(* Logix 5000 AddOnInstructionDefinition export HI6501_HMI_AOI_V1_2; software revision 30.00 *)

ADD_ON_INSTRUCTION HI6501_HMI_AOI_V1_2   (* revision 1.0 *)
VAR_IN_OUT
   From_Indicator : _0102:Hardy6500Series_3459222C:I:0; {required}   // Inputs from Hardy indicator
   To_Indicator : _0102:Hardy6500Series_B3FC222E:O:0; {required}   // Outputs to Hardy indicator
END_VAR
VAR_INPUT
   Remote_Zero : BOOL;   // Remote zero input signal
   Remote_Tare : BOOL;   // Remote tare input signal
   Mode_Select_PB : BOOL;   // Gross Net mode toggle select from faceplate
END_VAR
VAR_OUTPUT
   Gross_Mode_To_FP : BOOL; {access Read Only}   // Gross weight display mode output to faceplate
   Net_Mode_To_FP : BOOL; {access Read Only}   // Net weight display mode output to faceplate
   Gross_Weight : REAL; {access Read Only, visible}   // Gross weight
   Net_Weight : REAL; {access Read Only, visible}   // Net weight
   Alarm : BOOL; {access Read Only, visible}   // Alarm output
   Decimal_Point_To_FP : SINT;   // Decimal point parameter input value to faceplate
   Grads_To_FP : SINT;   // Graduations parameter input value to faceplate
   Unit_To_FP : SINT;   // Units parameter input value to faceplate
   Waversaver_To_FP : SINT;   // WAVERSAVER parameter input value to faceplate
   Num_Averages_To_FP : INT;   // Number of averages parameter input value to faceplate
   Loadcell_Sensitivity_To_FP : INT;   // Load cell sensitivity parameter input value to faceplate
   AutoZero_To_FP : INT;   // Auto zero parameter input value to faceplate
   AutoZero_Tol_To_FP : REAL;   // Auto zero tolerance parameter input value to faceplate
   Gravity_Correction_To_FP : REAL;   // Gravity correction parameter input value to faceplate
   Motion_Tol_To_FP : REAL;   // Motion tolerance parameter input value to faceplate
   Zero_Tol_To_FP : REAL;   // Zero tolerance parameter input value to faceplate
   Tare_Weight_To_FP : REAL;   // Tare weight parameter input value to faceplate
   Reference_Weight_To_FP : REAL;   // Reference weight parameter input value to faceplate
   Span_Weight_To_FP : REAL;   // Span weight parameter input value to faceplate
   Scale_Capacity_To_FP : REAL;   // Scale capacity parameter input value to faceplate
END_VAR
VAR_INPUT
   Read_Params_PB : BOOL;   // Read parameter command input from faceplate
   Save_PB : BOOL;   // Write parameter command input from faceplate
   Zero_PB : BOOL; {visible}   // Zero command from faceplate
   Tare_PB : BOOL; {visible}   // Tare command input from faceplate
   C2_Cal_PB : BOOL; {visible}   // C2 calibration command input from faceplate
   Cal_Low_PB : BOOL; {visible}   // Calibrate low command input from faceplate
   Cal_Hi_PB : BOOL; {visible}   // Calibrate high command input from faceplate
   Setup_PB : BOOL;   // Setup pushbutton parameter input to display Setup screen
   Params_PB : BOOL;   // Params pushbutton parameter input to display Parameters screen
   Filtering_PB : BOOL;   // Filtering pushbutton parameter input to display Filtering screen
   Calibration_PB : BOOL;   // Calibration pushbutton parameter input to display Calibration screen
   Home_PB : BOOL;   // Home pushbutton parameter input to display Home screen
   Traditional_Cal_PB : BOOL;   // Traditional Calibration pushbutton parameter input to display Traditional Calibration screen
   Auto_Zero_PB : BOOL;   // Auto Zero Enable/Disable pushbutton parameter input from faceplate
   Decimal_point_From_FP : SINT;   // Decimal point parameter output value from faceplate
   Grads_From_FP : SINT;   // Graduations parameter output value from faceplate
   Unit_From_FP : SINT;   // Units parameter output value from faceplate
   Waversaver_From_FP : SINT;   // WAVERSAVER parameter output value from faceplate
   Num_averages_From_FP : INT;   // Number of averages parameter output value from faceplate
   Loadcell_sensitivity_From_FP : INT;   // Load cell sensitivity parameter output value from faceplate
   AutoZero_From_FP : INT;   // Auto zero parameter output value from faceplate
   AutoZero_Tol_From_FP : REAL;   // Auto zero tloerance parameter output value from faceplate
   Gravity_correction_From_FP : REAL;   // Gravity correction parameter output value from faceplate
   Motion_Tol_From_FP : REAL;   // Motion tolerance parameter output value from faceplate
   Zero_Tol_From_FP : REAL;   // Zero tolerance parameter output value from faceplate
   Tare_Weight_From_FP : REAL;   // Tare weight parameter output value from faceplate
   Reference_Weight_From_FP : REAL;   // Reference weight parameter output value from faceplate
   Span_Weight_From_FP : REAL;   // Span weight parameter output value from faceplate to indicator
   Scale_Capacity_From_FP : REAL;   // Scale capacity parameter output value from faceplate
END_VAR
VAR_OUTPUT
   Cmd_Status_To_FP : INT; {access Read Only, visible}   // Command status output value to faceplate
   Instrument_Status_To_FP : INT; {access Read Only, visible}   // Instrument status output to faceplate
   Scale_Alarm : BOOL; {access Read Only}   // Scale error and alarm output bit to faceplate
   Status_Alarm : BOOL; {access Read Only}   // Status error and alarm bit output to faceplate
   Comm_Alarm : BOOL; {access Read Only}   // Communication error and alarm bit output to faceplate
   Display_Num : DINT; {access Read Only}   // Display number parameter value for faceplate animatiom
END_VAR
VAR_INPUT
   Decimal_Toggle_PB : BOOL;
END_VAR
VAR_OUTPUT
   GrossWtDecimal_To_FP : SINT; {access Read Only}
   NetWtDecimal_To_FP : SINT; {access Read Only}
END_VAR
VAR
   ZeroCmdSuccess : BOOL; {access None}
   Zero_Value : REAL; {access None}
   Zero_ONS : BOOL; {access None}
   Zero_Cmd : BOOL; {access None}
   WriteSpanWtSuccess : BOOL; {access None}
   WriteSpanWt_Cmd : BOOL; {access None}
   WriteRefWtSuccess : BOOL; {access None}
   WriteRefWt_Cmd : BOOL; {access None}
   Write_SpanWt_ONS : BOOL; {access None}
   Write_Delay_0 : TIMER := (PRE := 200); {access None}
   Write_Cmd_Sequencer : DINT; {access None}
   Test_Counter : COUNTER; {access None}
   TareCmdSuccess : BOOL; {access None}
   Tare_ONS : BOOL; {access None}
   Tare_Cmd : BOOL; {access None}
   SpanWtDelay_Timer : TIMER := (PRE := 111); {access None}
   SpanWtClearDelay_Timer : TIMER := (PRE := 111); {access None}
   SpanWt_Success_ONS : BOOL; {access None}
   Span_Wt_FLOAT_Monitor : REAL; {access None}
   Save_PB_ONS : BOOL; {access None}
   RefWtDelay_Timer : TIMER := (PRE := 111); {access None}
   RefWtClearDelay_Timer : TIMER := (PRE := 111); {access None}
   RefWt_Success_ONS : BOOL; {access None}
   ReadUnitsSuccess : BOOL; {access None}
   ReadUnits_Cmd : BOOL; {access None}
   ReadSpanWeightSuccess : BOOL; {access None}
   ReadSpanWeight_Cmd : BOOL; {access None}
   ReadRefWeightSuccess : BOOL; {access None}
   ReadRefWeight_Cmd : BOOL; {access None}
   ReadLoadCellSensSuccess : BOOL; {access None}
   ReadLoadCellSens_Cmd : BOOL; {access None}
   ReadGravityCorrectSuccess : BOOL; {access None}
   ReadGravityCorrection_Cmd : BOOL; {access None}
   ReadGradsSuccess : BOOL; {access None}
   ReadGrads_Cmd : BOOL; {access None}
   ReadDecimalPtSuccess : BOOL; {access None}
   ReadDecimalPt_Cmd : BOOL; {access None}
   Read_Params_PB_ONS : BOOL; {access None}
   Read_Delay_4 : TIMER := (PRE := 111); {access None}
   Read_Delay_3 : TIMER := (PRE := 111); {access None}
   Read_Delay_2 : TIMER := (PRE := 111); {access None}
   Read_Delay_1 : TIMER := (PRE := 111); {access None}
   Read_Delay_0 : TIMER := (PRE := 111); {access None}
   PlaceHolder : BOOL; {access None}
   ParameterResetTimer : TIMER := (PRE := 3000); {access None}
   ModeCounter : COUNTER := (PRE := 2); {access None}
   Mode_ONS1 : BOOL; {access None}
   InstrumentStatus : INT; {access None}
   HeartbeatCapture : INT; {access None}
   HeartbeatCaptureTimer : TIMER := (PRE := 250); {access None}
   HeartbeatAlarmTimer : TIMER := (PRE := 1000); {access None}
   Heartbeat : INT; {access None}
   CmdStatus : INT; {access None}
   DecimalPtDelay_Timer : TIMER := (PRE := 111); {access None}
   DecimalPtClearDelay_Timer : TIMER := (PRE := 111); {access None}
   DecimalCounter : COUNTER := (PRE := 3); {access None}
   Decimal_Toggle_ONS2 : BOOL; {access None}
   Decimal_Toggle_ONS1 : BOOL; {access None}
   CmdEcho : INT; {access None}
   CalLowCmdSuccess : BOOL; {access None}
   CalLow_ONS : BOOL; {access None}
   CalLow_Cmd : BOOL; {access None}
   CalHiCmdSuccess : BOOL; {access None}
   CalHI_ONS : BOOL; {access None}
   CalHi_Cmd : BOOL; {access None}
   C2CalCmdSuccess : BOOL; {access None}
   C2Cal_ONS : BOOL; {access None}
   C2Cal_Cmd : BOOL; {access None}
END_VAR

ROUTINE Logic   (* ladder *)
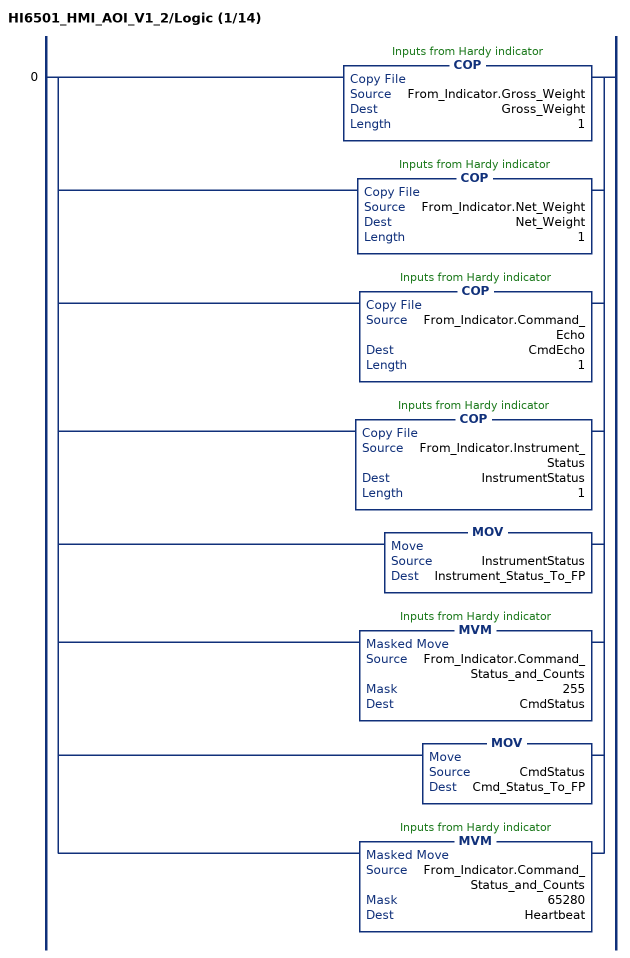
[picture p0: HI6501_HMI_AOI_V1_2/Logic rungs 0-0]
   0: [COP(From_Indicator.Gross_Weight,Gross_Weight,1) ,COP(From_Indicator.Net_Weight,Net_Weight,1) ,COP(From_Indicator.Command_Echo,CmdEcho,1) ,COP(From_Indicator.Instrument_Status,InstrumentStatus,1) ,MOV(InstrumentStatus,Instrument_Status_To_FP) ,MVM(From_Indicator.Command_Status_and_Counts,255,CmdStatus) ,MOV(CmdStatus,Cmd_Status_To_FP) ,MVM(From_Indicator.Command_Status_and_Counts,65280,Heartbeat) ];
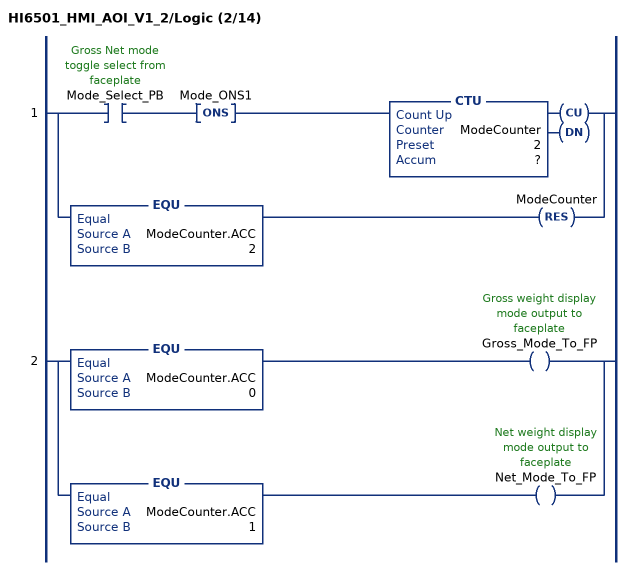
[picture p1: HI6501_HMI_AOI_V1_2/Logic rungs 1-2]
   1: [XIC(Mode_Select_PB) ONS(Mode_ONS1) CTU(ModeCounter,?,?) ,EQU(ModeCounter.ACC,2) RES(ModeCounter) ];
   2: [EQU(ModeCounter.ACC,0) OTE(Gross_Mode_To_FP) ,EQU(ModeCounter.ACC,1) OTE(Net_Mode_To_FP) ];
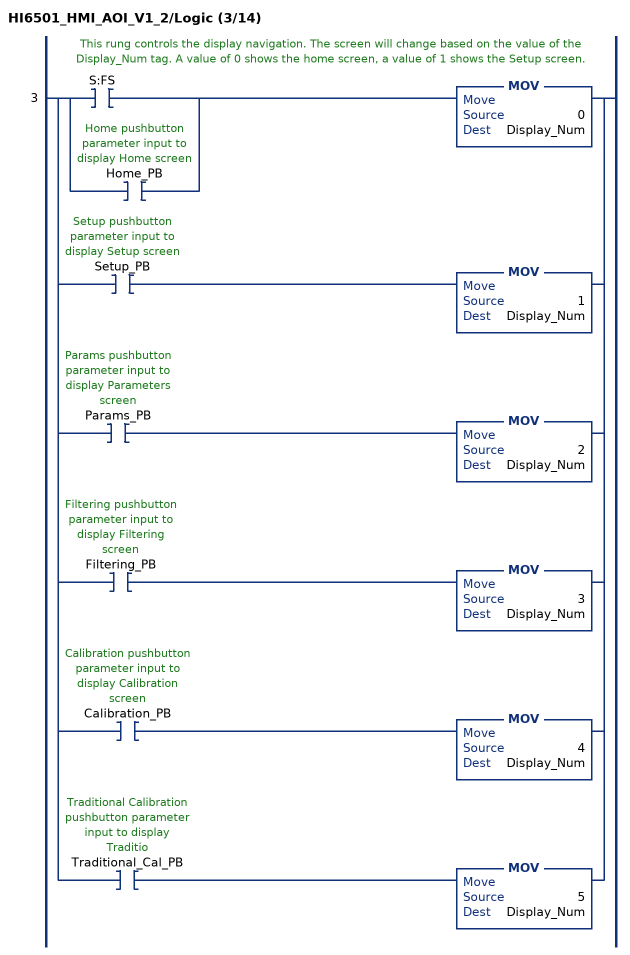
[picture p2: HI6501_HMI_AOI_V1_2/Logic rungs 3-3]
   // This rung controls the display navigation. The screen will change based on the value of the Display_Num tag. A value of 0 shows the home screen, a value of 1 shows the Setup screen.
   3: [[XIC(S:FS) ,XIC(Home_PB) ] MOV(0,Display_Num) ,XIC(Setup_PB) MOV(1,Display_Num) ,XIC(Params_PB) MOV(2,Display_Num) ,XIC(Filtering_PB) MOV(3,Display_Num) ,XIC(Calibration_PB) MOV(4,Display_Num) ,XIC(Traditional_Cal_PB) MOV(5,Display_Num) ];
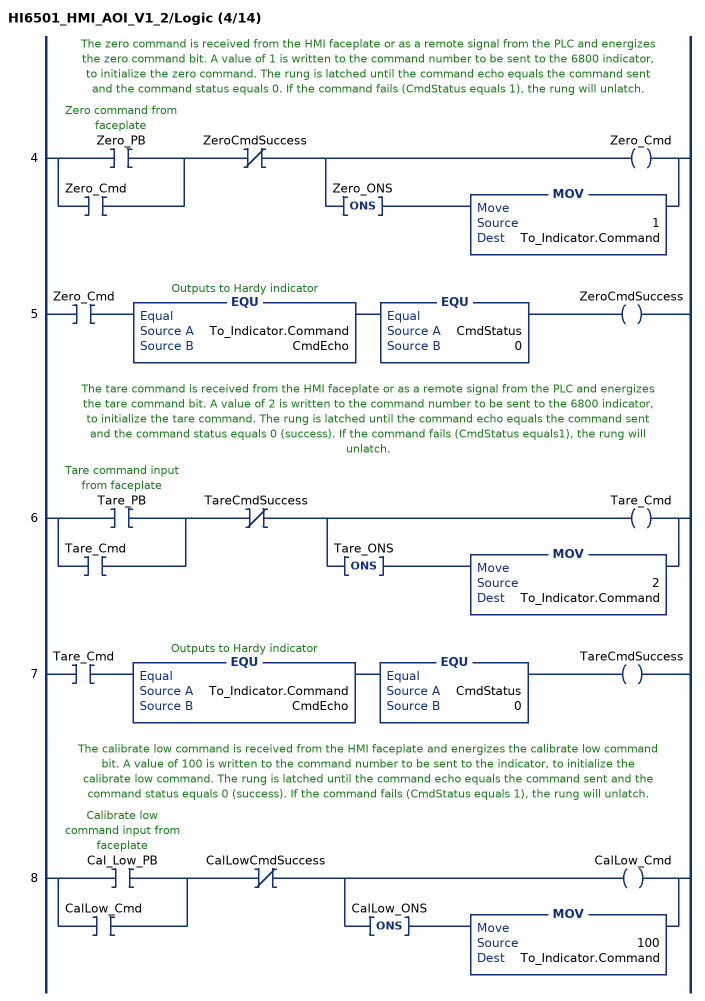
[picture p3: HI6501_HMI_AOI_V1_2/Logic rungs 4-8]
   // The zero command is received from the HMI faceplate or as a remote signal from the PLC and energizes the zero command bit. A value of 1 is written to the command number to be sent to the 6800 indicator, to initialize the zero command. The rung is latched until the command echo equals the command sent and the command status equals 0. If the command fails (CmdStatus equals 1), the rung will unlatch.
   4: [XIC(Zero_PB) ,XIC(Zero_Cmd) ]XIO(ZeroCmdSuccess)[OTE(Zero_Cmd) ,ONS(Zero_ONS) MOV(1,To_Indicator.Command) ];
   5: XIC(Zero_Cmd)EQU(To_Indicator.Command,CmdEcho)EQU(CmdStatus,0)OTE(ZeroCmdSuccess);
   // The tare command is received from the HMI faceplate or as a remote signal from the PLC and energizes the tare command bit. A value of 2 is written to the command number to be sent to the 6800 indicator, to initialize the tare command. The rung is latched until the command echo equals the command sent and the command status equals 0 (success). If the command fails (CmdStatus equals1), the rung will unlatch.
   6: [XIC(Tare_PB) ,XIC(Tare_Cmd) ]XIO(TareCmdSuccess)[OTE(Tare_Cmd) ,ONS(Tare_ONS) MOV(2,To_Indicator.Command) ];
   7: XIC(Tare_Cmd)EQU(To_Indicator.Command,CmdEcho)EQU(CmdStatus,0)OTE(TareCmdSuccess);
   // The calibrate low command is received from the HMI faceplate and energizes the calibrate low command bit. A value of 100 is written to the command number to be sent to the indicator, to initialize the calibrate low command. The rung is latched until the command echo equals the command sent and the command status equals 0 (success). If the command fails (CmdStatus equals 1), the rung will unlatch.
   8: [XIC(Cal_Low_PB) ,XIC(CalLow_Cmd) ]XIO(CalLowCmdSuccess)[OTE(CalLow_Cmd) ,ONS(CalLow_ONS) MOV(100,To_Indicator.Command) ];
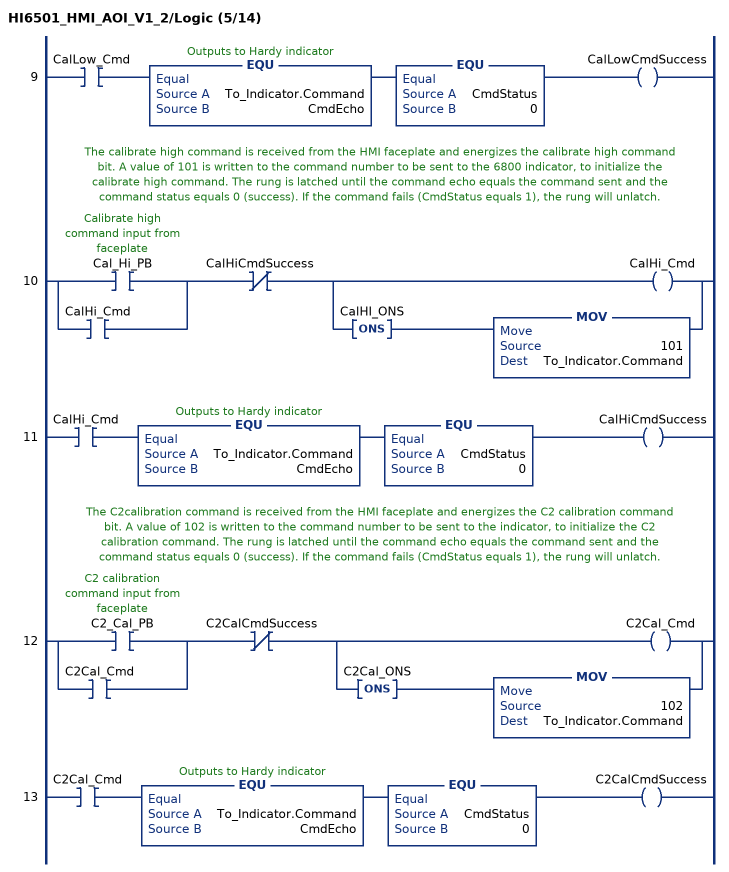
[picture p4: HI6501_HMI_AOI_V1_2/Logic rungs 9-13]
   9: XIC(CalLow_Cmd)EQU(To_Indicator.Command,CmdEcho)EQU(CmdStatus,0)OTE(CalLowCmdSuccess);
   // The calibrate high command is received from the HMI faceplate and energizes the calibrate high command bit. A value of 101 is written to the command number to be sent to the 6800 indicator, to initialize the calibrate high command. The rung is latched until the command echo equals the command sent and the command status equals 0 (success). If the command fails (CmdStatus equals 1), the rung will unlatch.
   10: [XIC(Cal_Hi_PB) ,XIC(CalHi_Cmd) ]XIO(CalHiCmdSuccess)[OTE(CalHi_Cmd) ,ONS(CalHI_ONS) MOV(101,To_Indicator.Command) ];
   11: XIC(CalHi_Cmd)EQU(To_Indicator.Command,CmdEcho)EQU(CmdStatus,0)OTE(CalHiCmdSuccess);
   // The C2calibration command is received from the HMI faceplate and energizes the C2 calibration command bit. A value of 102 is written to the command number to be sent to the indicator, to initialize the C2 calibration command. The rung is latched until the command echo equals the command sent and the command status equals 0 (success). If the command fails (CmdStatus equals 1), the rung will unlatch.
   12: [XIC(C2_Cal_PB) ,XIC(C2Cal_Cmd) ]XIO(C2CalCmdSuccess)[OTE(C2Cal_Cmd) ,ONS(C2Cal_ONS) MOV(102,To_Indicator.Command) ];
   13: XIC(C2Cal_Cmd)EQU(To_Indicator.Command,CmdEcho)EQU(CmdStatus,0)OTE(C2CalCmdSuccess);
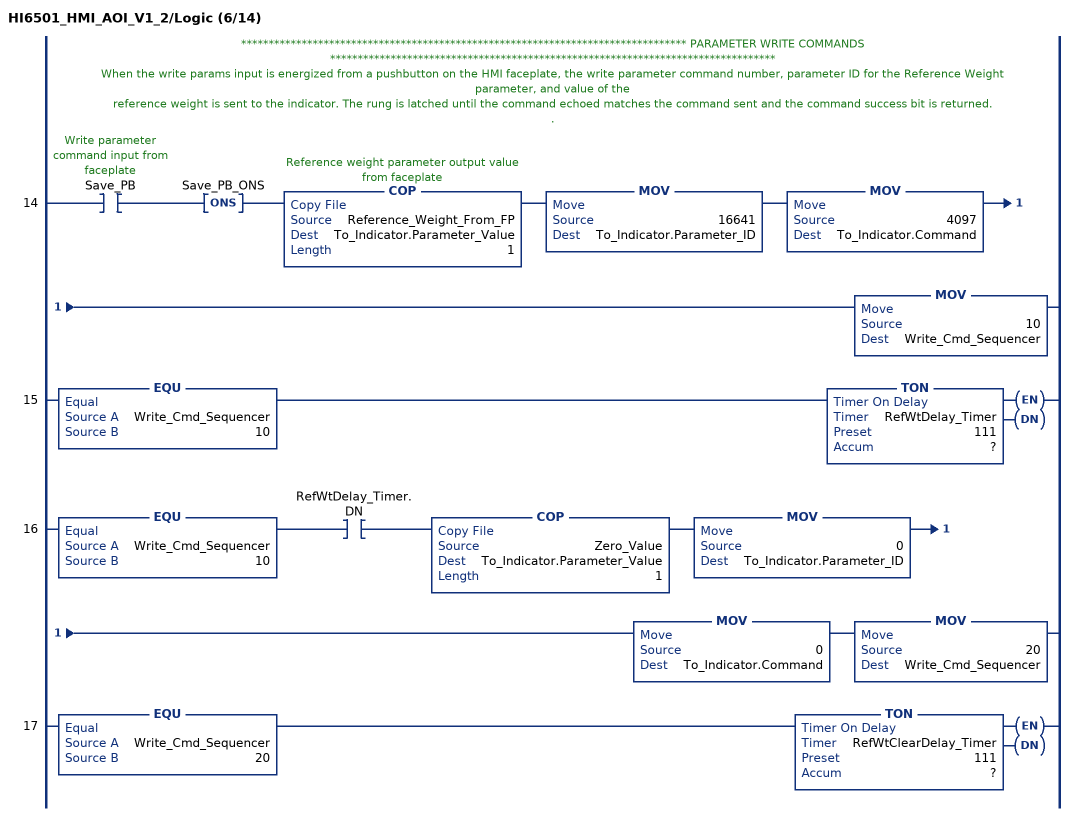
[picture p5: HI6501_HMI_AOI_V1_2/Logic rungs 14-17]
   // ********************************************************************************* PARAMETER WRITE COMMANDS *********************************************************************************
   // When the write params input is energized from a pushbutton on the HMI faceplate, the write parameter command number, parameter ID for the Reference Weight parameter, and value of the
   // reference weight is sent to the indicator. The rung is latched until the command echoed matches the command sent and the command success bit is returned.
   // .
   14: XIC(Save_PB)ONS(Save_PB_ONS)COP(Reference_Weight_From_FP,To_Indicator.Parameter_Value,1)MOV(16641,To_Indicator.Parameter_ID)MOV(4097,To_Indicator.Command)MOV(10,Write_Cmd_Sequencer);
   15: EQU(Write_Cmd_Sequencer,10)TON(RefWtDelay_Timer,?,?);
   16: EQU(Write_Cmd_Sequencer,10)XIC(RefWtDelay_Timer.DN)COP(Zero_Value,To_Indicator.Parameter_Value,1)MOV(0,To_Indicator.Parameter_ID)MOV(0,To_Indicator.Command)MOV(20,Write_Cmd_Sequencer);
   17: EQU(Write_Cmd_Sequencer,20)TON(RefWtClearDelay_Timer,?,?);
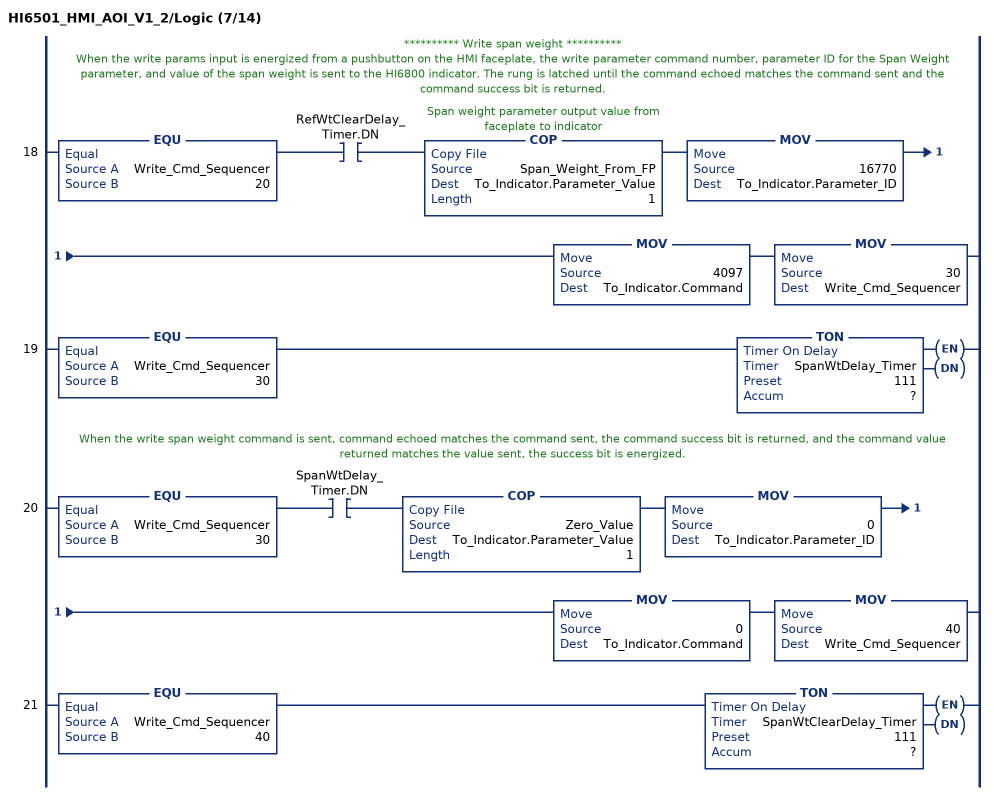
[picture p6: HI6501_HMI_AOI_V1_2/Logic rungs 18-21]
   // ********** Write span weight **********
   // When the write params input is energized from a pushbutton on the HMI faceplate, the write parameter command number, parameter ID for the Span Weight parameter, and value of the span weight is sent to the HI6800 indicator. The rung is latched until the command echoed matches the command sent and the command success bit is returned.
   18: EQU(Write_Cmd_Sequencer,20)XIC(RefWtClearDelay_Timer.DN)COP(Span_Weight_From_FP,To_Indicator.Parameter_Value,1)MOV(16770,To_Indicator.Parameter_ID)MOV(4097,To_Indicator.Command)MOV(30,Write_Cmd_Sequencer);
   19: EQU(Write_Cmd_Sequencer,30)TON(SpanWtDelay_Timer,?,?);
   // When the write span weight command is sent, command echoed matches the command sent, the command success bit is returned, and the command value returned matches the value sent, the success bit is energized.
   20: EQU(Write_Cmd_Sequencer,30)XIC(SpanWtDelay_Timer.DN)COP(Zero_Value,To_Indicator.Parameter_Value,1)MOV(0,To_Indicator.Parameter_ID)MOV(0,To_Indicator.Command)MOV(40,Write_Cmd_Sequencer);
   21: EQU(Write_Cmd_Sequencer,40)TON(SpanWtClearDelay_Timer,?,?);
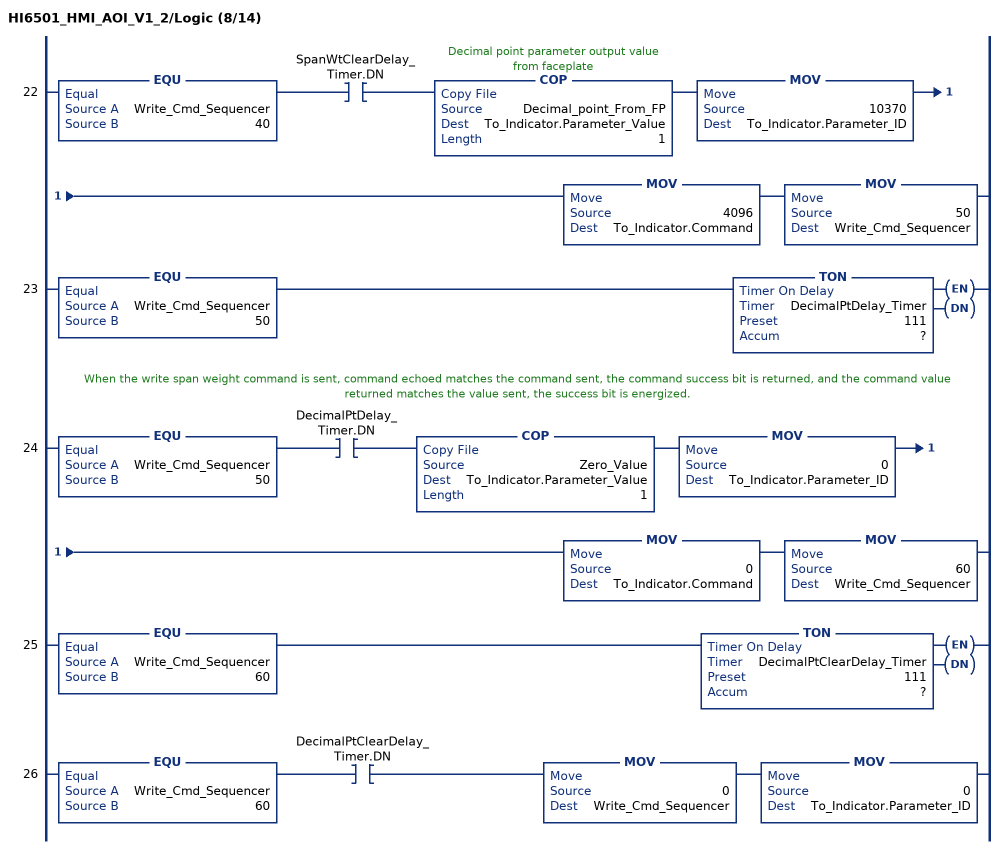
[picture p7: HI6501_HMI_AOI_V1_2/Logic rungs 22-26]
   22: EQU(Write_Cmd_Sequencer,40)XIC(SpanWtClearDelay_Timer.DN)COP(Decimal_point_From_FP,To_Indicator.Parameter_Value,1)MOV(10370,To_Indicator.Parameter_ID)MOV(4096,To_Indicator.Command)MOV(50,Write_Cmd_Sequencer);
   23: EQU(Write_Cmd_Sequencer,50)TON(DecimalPtDelay_Timer,?,?);
   // When the write span weight command is sent, command echoed matches the command sent, the command success bit is returned, and the command value returned matches the value sent, the success bit is energized.
   24: EQU(Write_Cmd_Sequencer,50)XIC(DecimalPtDelay_Timer.DN)COP(Zero_Value,To_Indicator.Parameter_Value,1)MOV(0,To_Indicator.Parameter_ID)MOV(0,To_Indicator.Command)MOV(60,Write_Cmd_Sequencer);
   25: EQU(Write_Cmd_Sequencer,60)TON(DecimalPtClearDelay_Timer,?,?);
   26: EQU(Write_Cmd_Sequencer,60)XIC(DecimalPtClearDelay_Timer.DN)MOV(0,Write_Cmd_Sequencer)MOV(0,To_Indicator.Parameter_ID);
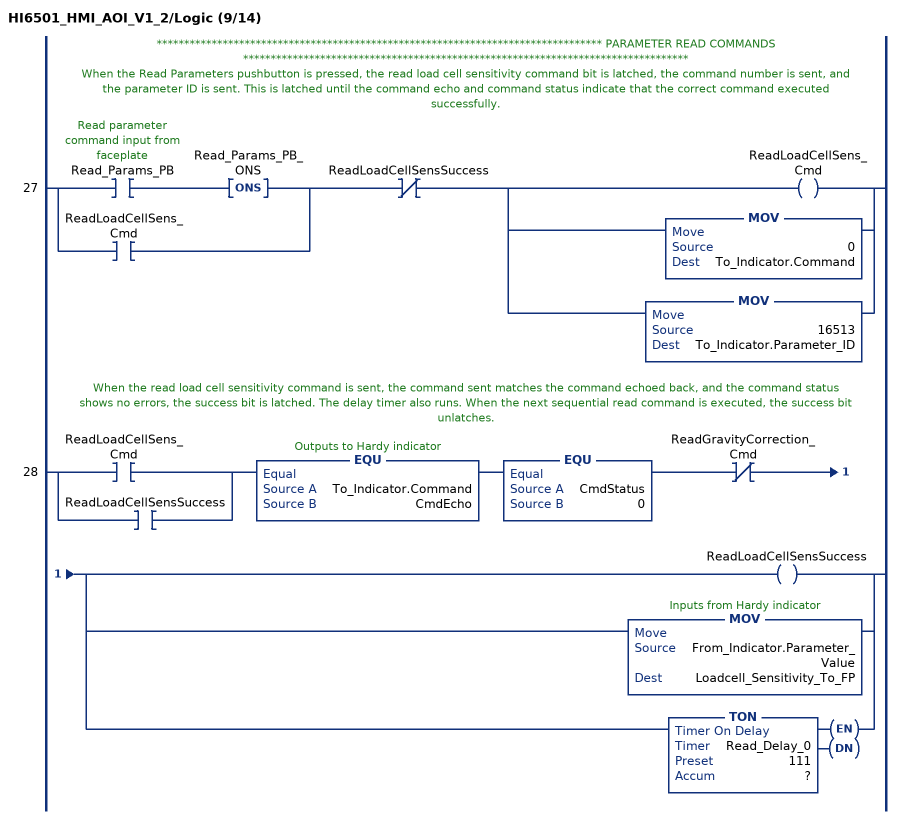
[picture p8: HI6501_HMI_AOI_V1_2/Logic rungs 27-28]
   // ********************************************************************************* PARAMETER READ COMMANDS *********************************************************************************
   // When the Read Parameters pushbutton is pressed, the read load cell sensitivity command bit is latched, the command number is sent, and the parameter ID is sent. This is latched until the command echo and command status indicate that the correct command executed successfully.
   27: [XIC(Read_Params_PB) ONS(Read_Params_PB_ONS) ,XIC(ReadLoadCellSens_Cmd) ]XIO(ReadLoadCellSensSuccess)[OTE(ReadLoadCellSens_Cmd) ,MOV(0,To_Indicator.Command) ,MOV(16513,To_Indicator.Parameter_ID) ];
   // When the read load cell sensitivity command is sent, the command sent matches the command echoed back, and the command status shows no errors, the success bit is latched. The delay timer also runs. When the next sequential read command is executed, the success bit unlatches.
   28: [XIC(ReadLoadCellSens_Cmd) ,XIC(ReadLoadCellSensSuccess) ]EQU(To_Indicator.Command,CmdEcho)EQU(CmdStatus,0)XIO(ReadGravityCorrection_Cmd)[OTE(ReadLoadCellSensSuccess) ,MOV(From_Indicator.Parameter_Value,Loadcell_Sensitivity_To_FP) ,TON(Read_Delay_0,?,?) ];
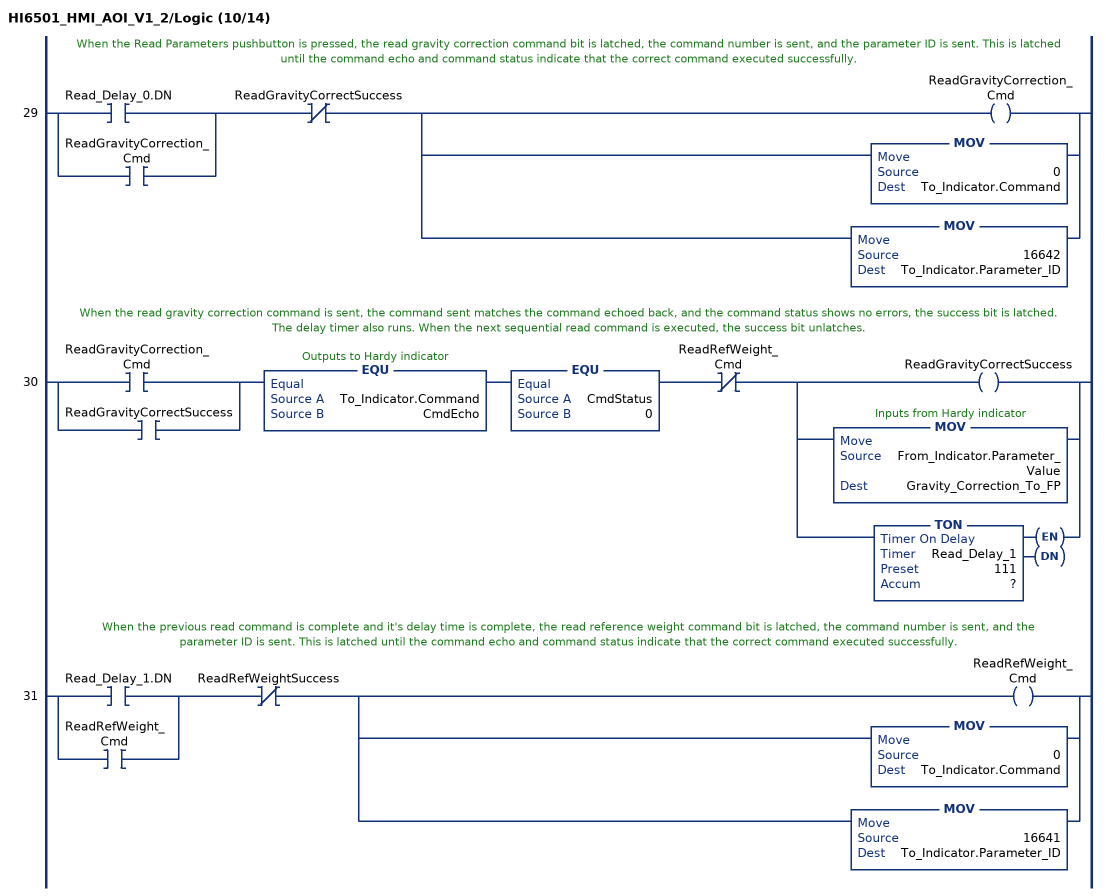
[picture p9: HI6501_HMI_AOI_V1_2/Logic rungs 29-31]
   // When the Read Parameters pushbutton is pressed, the read gravity correction command bit is latched, the command number is sent, and the parameter ID is sent. This is latched until the command echo and command status indicate that the correct command executed successfully.
   29: [XIC(Read_Delay_0.DN) ,XIC(ReadGravityCorrection_Cmd) ]XIO(ReadGravityCorrectSuccess)[OTE(ReadGravityCorrection_Cmd) ,MOV(0,To_Indicator.Command) ,MOV(16642,To_Indicator.Parameter_ID) ];
   // When the read gravity correction command is sent, the command sent matches the command echoed back, and the command status shows no errors, the success bit is latched. The delay timer also runs. When the next sequential read command is executed, the success bit unlatches.
   30: [XIC(ReadGravityCorrection_Cmd) ,XIC(ReadGravityCorrectSuccess) ]EQU(To_Indicator.Command,CmdEcho)EQU(CmdStatus,0)XIO(ReadRefWeight_Cmd)[OTE(ReadGravityCorrectSuccess) ,MOV(From_Indicator.Parameter_Value,Gravity_Correction_To_FP) ,TON(Read_Delay_1,?,?) ];
   // When the previous read command is complete and it's delay time is complete, the read reference weight command bit is latched, the command number is sent, and the parameter ID is sent. This is latched until the command echo and command status indicate that the correct command executed successfully.
   31: [XIC(Read_Delay_1.DN) ,XIC(ReadRefWeight_Cmd) ]XIO(ReadRefWeightSuccess)[OTE(ReadRefWeight_Cmd) ,MOV(0,To_Indicator.Command) ,MOV(16641,To_Indicator.Parameter_ID) ];
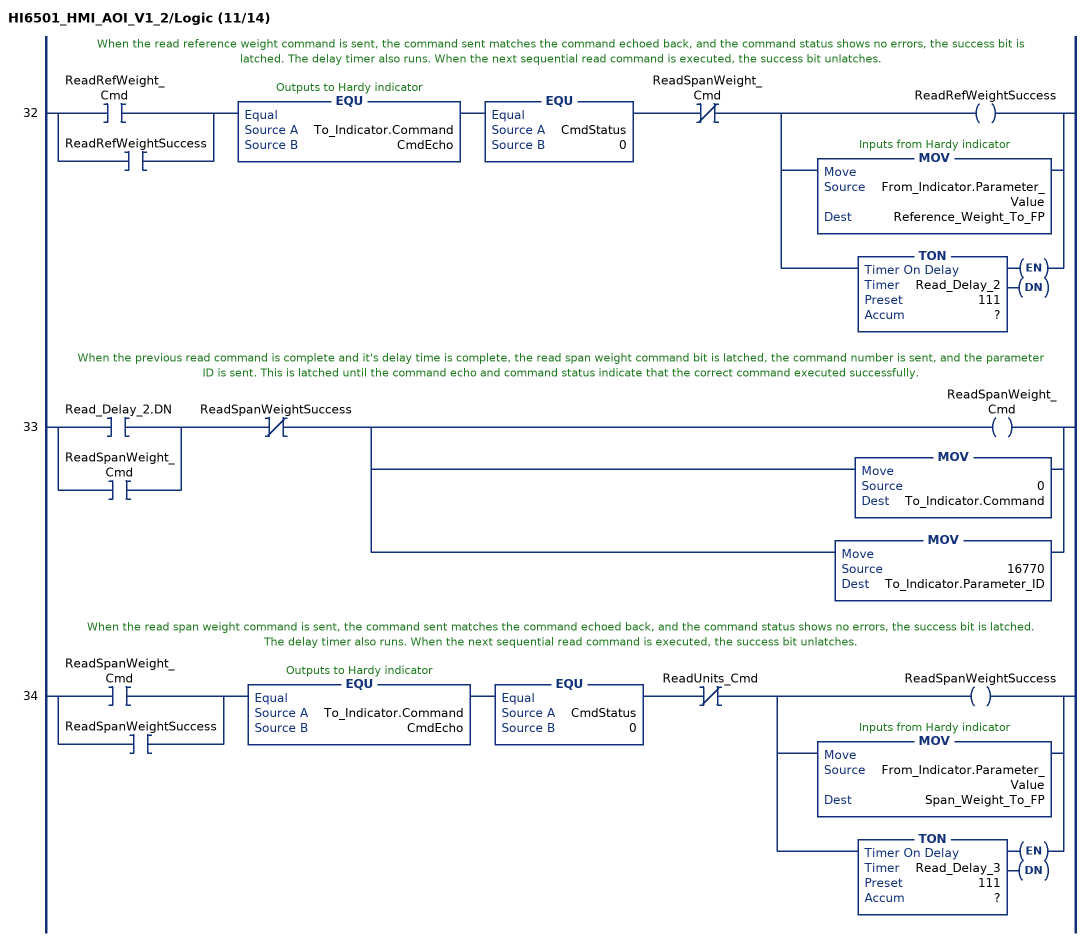
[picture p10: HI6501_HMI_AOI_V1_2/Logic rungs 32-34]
   // When the read reference weight command is sent, the command sent matches the command echoed back, and the command status shows no errors, the success bit is latched. The delay timer also runs. When the next sequential read command is executed, the success bit unlatches.
   32: [XIC(ReadRefWeight_Cmd) ,XIC(ReadRefWeightSuccess) ]EQU(To_Indicator.Command,CmdEcho)EQU(CmdStatus,0)XIO(ReadSpanWeight_Cmd)[OTE(ReadRefWeightSuccess) ,MOV(From_Indicator.Parameter_Value,Reference_Weight_To_FP) ,TON(Read_Delay_2,?,?) ];
   // When the previous read command is complete and it's delay time is complete, the read span weight command bit is latched, the command number is sent, and the parameter ID is sent. This is latched until the command echo and command status indicate that the correct command executed successfully.
   33: [XIC(Read_Delay_2.DN) ,XIC(ReadSpanWeight_Cmd) ]XIO(ReadSpanWeightSuccess)[OTE(ReadSpanWeight_Cmd) ,MOV(0,To_Indicator.Command) ,MOV(16770,To_Indicator.Parameter_ID) ];
   // When the read span weight command is sent, the command sent matches the command echoed back, and the command status shows no errors, the success bit is latched. The delay timer also runs. When the next sequential read command is executed, the success bit unlatches.
   34: [XIC(ReadSpanWeight_Cmd) ,XIC(ReadSpanWeightSuccess) ]EQU(To_Indicator.Command,CmdEcho)EQU(CmdStatus,0)XIO(ReadUnits_Cmd)[OTE(ReadSpanWeightSuccess) ,MOV(From_Indicator.Parameter_Value,Span_Weight_To_FP) ,TON(Read_Delay_3,?,?) ];
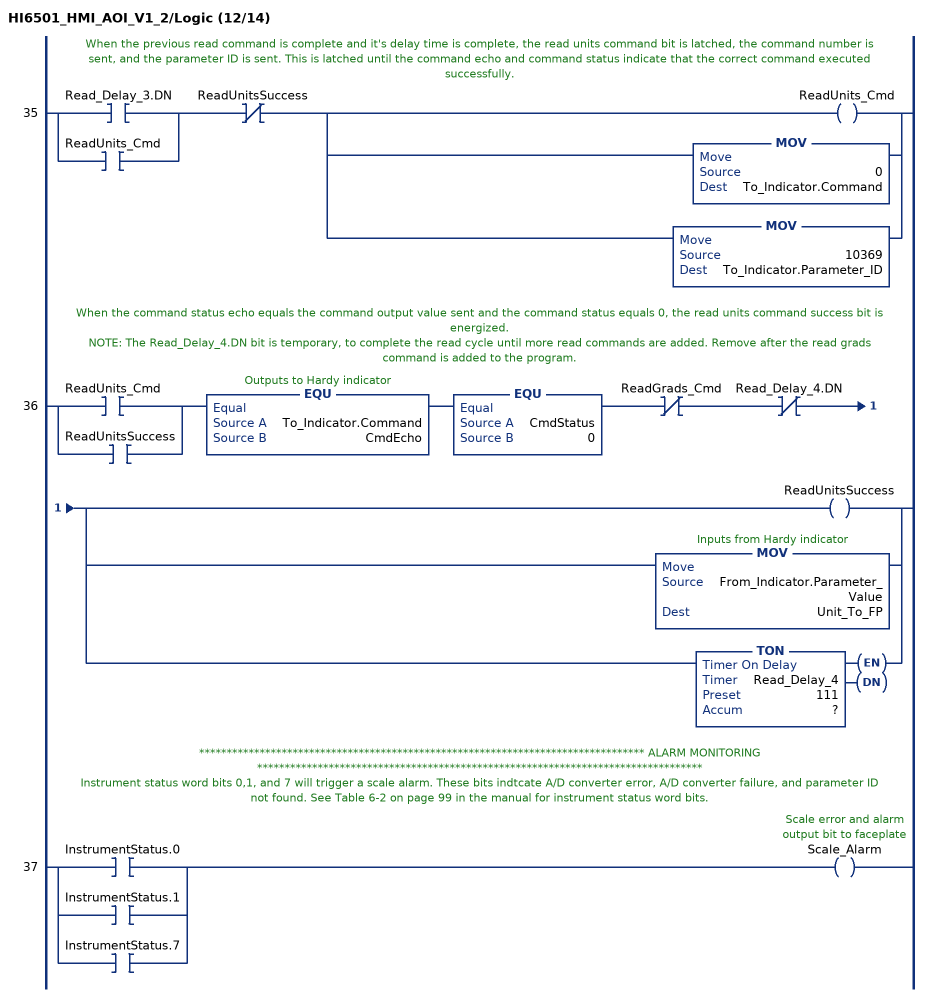
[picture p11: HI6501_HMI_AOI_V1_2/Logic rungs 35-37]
   // When the previous read command is complete and it's delay time is complete, the read units command bit is latched, the command number is sent, and the parameter ID is sent. This is latched until the command echo and command status indicate that the correct command executed successfully.
   35: [XIC(Read_Delay_3.DN) ,XIC(ReadUnits_Cmd) ]XIO(ReadUnitsSuccess)[OTE(ReadUnits_Cmd) ,MOV(0,To_Indicator.Command) ,MOV(10369,To_Indicator.Parameter_ID) ];
   // When the command status echo equals the command output value sent and the command status equals 0, the read units command success bit is energized.
   // NOTE: The Read_Delay_4.DN bit is temporary, to complete the read cycle until more read commands are added. Remove after the read grads command is added to the program.
   36: [XIC(ReadUnits_Cmd) ,XIC(ReadUnitsSuccess) ]EQU(To_Indicator.Command,CmdEcho)EQU(CmdStatus,0)XIO(ReadGrads_Cmd)XIO(Read_Delay_4.DN)[OTE(ReadUnitsSuccess) ,MOV(From_Indicator.Parameter_Value,Unit_To_FP) ,TON(Read_Delay_4,?,?) ];
   // ********************************************************************************* ALARM MONITORING *********************************************************************************
   // Instrument status word bits 0,1, and 7 will trigger a scale alarm. These bits indtcate A/D converter error, A/D converter failure, and parameter ID not found. See Table 6-2 on page 99 in the manual for instrument status word bits.
   37: [XIC(InstrumentStatus.0) ,XIC(InstrumentStatus.1) ,XIC(InstrumentStatus.7) ]OTE(Scale_Alarm);
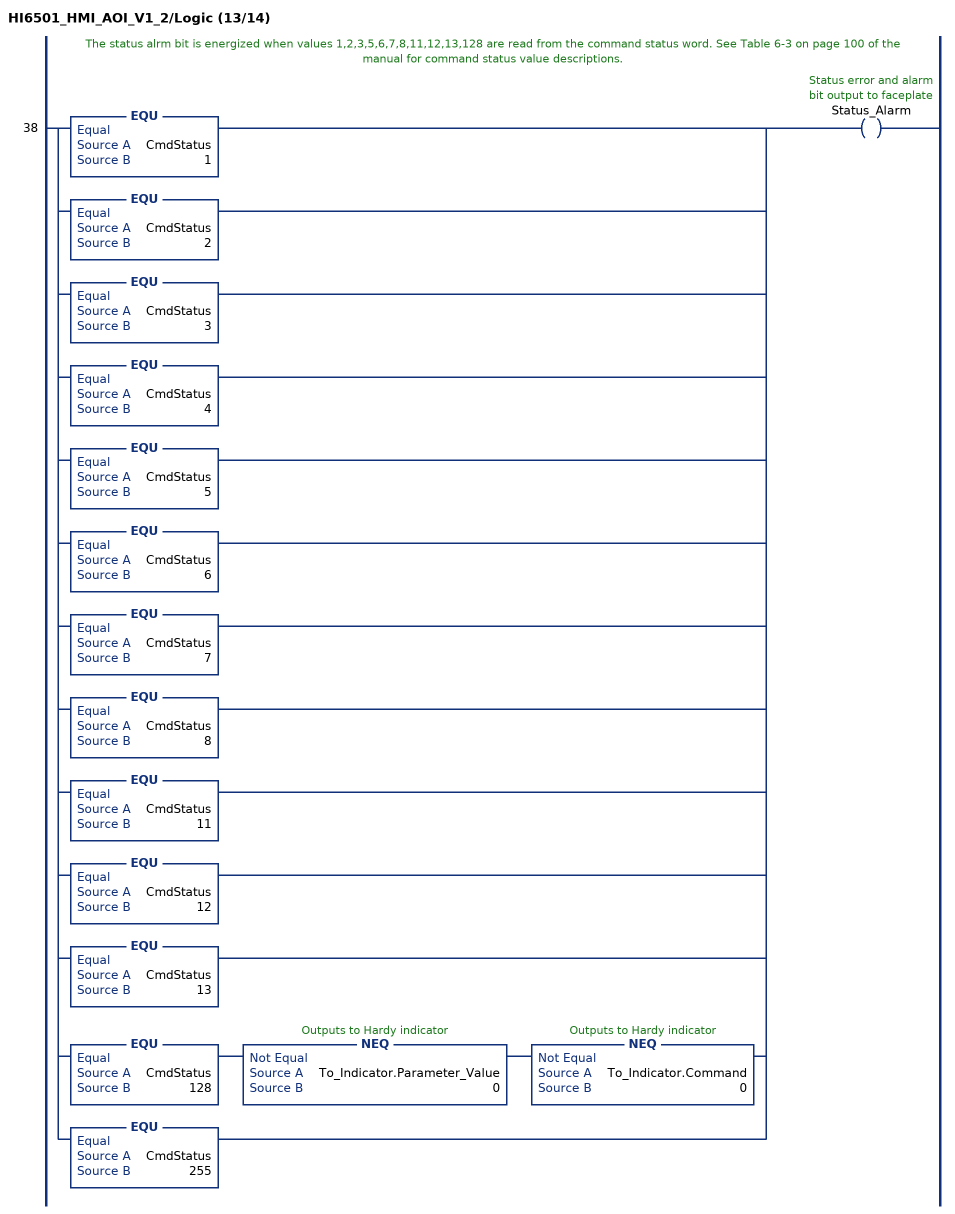
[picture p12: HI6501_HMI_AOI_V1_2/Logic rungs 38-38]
   // The status alrm bit is energized when values 1,2,3,5,6,7,8,11,12,13,128 are read from the command status word. See Table 6-3 on page 100 of the manual for command status value descriptions.
   38: [EQU(CmdStatus,1) ,EQU(CmdStatus,2) ,EQU(CmdStatus,3) ,EQU(CmdStatus,4) ,EQU(CmdStatus,5) ,EQU(CmdStatus,6) ,EQU(CmdStatus,7) ,EQU(CmdStatus,8) ,EQU(CmdStatus,11) ,EQU(CmdStatus,12) ,EQU(CmdStatus,13) ,EQU(CmdStatus,128) NEQ(To_Indicator.Parameter_Value,0) NEQ(To_Indicator.Command,0) ,EQU(CmdStatus,255) ]OTE(Status_Alarm);
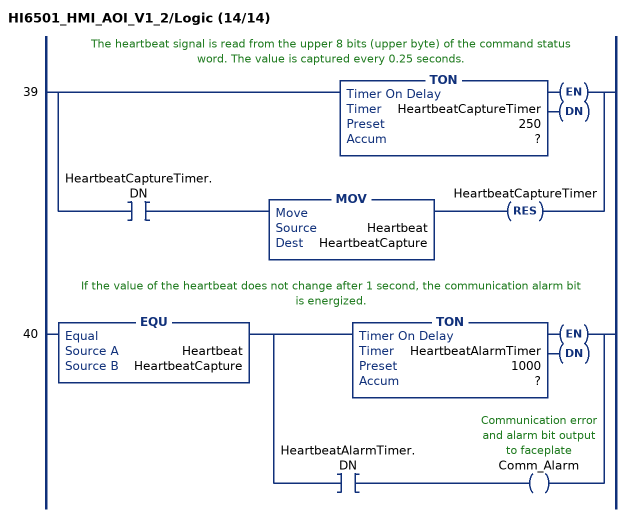
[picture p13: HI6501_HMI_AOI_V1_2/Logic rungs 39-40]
   // The heartbeat signal is read from the upper 8 bits (upper byte) of the command status word. The value is captured every 0.25 seconds.
   39: [TON(HeartbeatCaptureTimer,?,?) ,XIC(HeartbeatCaptureTimer.DN) MOV(Heartbeat,HeartbeatCapture) RES(HeartbeatCaptureTimer) ];
   // If the value of the heartbeat does not change after 1 second, the communication alarm bit is energized.
   40: EQU(Heartbeat,HeartbeatCapture)[TON(HeartbeatAlarmTimer,?,?) ,XIC(HeartbeatAlarmTimer.DN) OTE(Comm_Alarm) ];
END_ROUTINE
END_ADD_ON_INSTRUCTION
